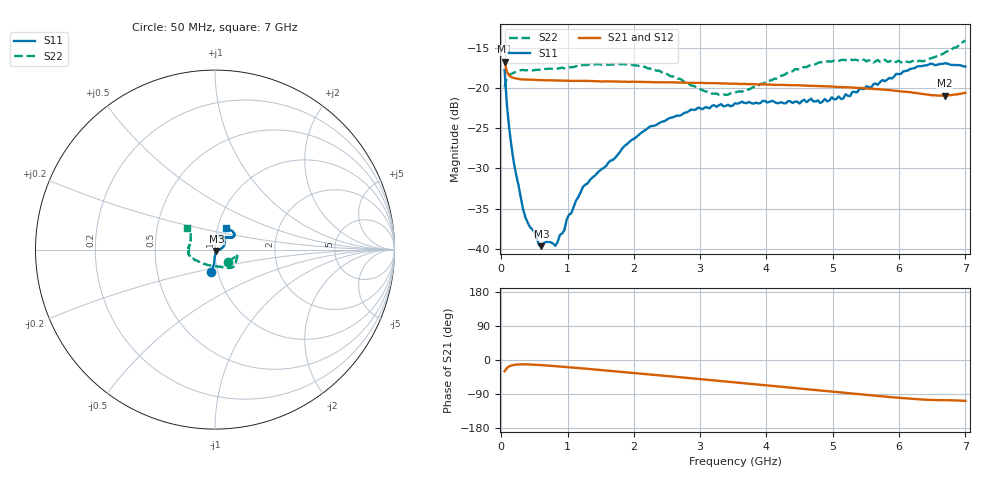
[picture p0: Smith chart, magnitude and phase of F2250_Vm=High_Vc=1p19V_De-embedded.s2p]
! Integrated Device Technology
! Corporate Headquarters
! 6024 Silver Creek Valley Road
! San Jose, CA 95138  USA
! Phone:  1-408-284-8200
! Toll Free:  1-800-223-1366
! Webpage:  http://www.idt.com/
! Timing and RF Division
! 515 Groton Road, Suite 102
! Westford, MA 01886-6024
! Device:  F2250
! Description: Voltage Variable RF Attenuator
! Frequency:  50.0 -  6000.00 MHz
! Package:  3x3 mm Thin QFN Plastic Package: 16 pin
! Ports:  2 RF, 3 DC
!  Pin  1  = GND
!  Pin  2  = NC
!  Pin  3  = RF1  = Port 1
!  Pin  4  = NC
!  Pin  5  = GND
!  Pin  6  = GND
!  Pin  7  = GND
!  Pin  8  = GND
!  Pin  9  = NC
!  Pin 10  = RF2  = Port 2
!  Pin 11  = NC
!  Pin 12  = GND
!  Pin 13  = GND
!  Pin 14  = VCNTRL
!  Pin 15  = VDD
!  Pin 16  = VMODE
! Vcntrl:  1.190 Volts
! Vmode:  +3.300 Volts
! Vdd:  +3.30  Volts
! Current:  1.330 mA
! Data:  The device was measured on a the F2250 evaluation board which has
!  individual transmission lines to the RF pins.  Data was collected
!  using a calibrated network analyzer.  The evaluation board was
!  de-embedded using a TRL calibration technique.
!  The reference plane is the edge of the package pin.
! Misc:  SN 10
!  Action Tracker AT0258
! Date Measured:  2014-11-26
! Date:  2015-10-15  MJV
! Note:
!  Integrated Device Technology supplies this data as a sample of measured
!  data at the package pin for this product.  Your particular data for this
!  product may vary.
!  Data was taken at 25 degrees C.
!  Integrated Device Technology reserves the right to change this data at anytime.
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# GHz S dB R 50
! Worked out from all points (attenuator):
!   201 points, 50 MHz to 7 GHz, reference 50 ohm
!   highest |S21| = -16.75 dB at 50 MHz (marker M1); lowest = -21.0 dB at 6.687 GHz (marker M2)
!   lowest |S11| = -39.6 dB at 606 MHz (marker M3), VSWR 1.02, Z = 50.7 - j0.741 ohm
!   |S11| at or under -10 dB: start of sweep to end of sweep
!   |S22| runs from -20.9 to -14.1 dB; largest |S21 - S12| = 0.00038
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0.05  -17.78 -99.8  -16.75 -29.8  -16.73 -29.8  -19.93 -42.3
0.08475  -22.13 -93.7  -18.02 -21.2  -18.02 -21.2  -18.62 -20.7
0.15425  -27.31 -92.7  -18.68 -14.4  -18.67 -14.4  -18.27 -13.0
0.189  -29.28 -90.4  -18.78 -13.0  -18.77 -13.0  -18.11 -12.4
0.328  -35.03 -76.1  -18.95 -11.4  -18.94 -11.4  -17.79 -12.8
0.43225  -37.28 -73.6  -18.98 -11.8  -19.00 -11.8  -17.83 -13.9
0.606  -39.64 -44.5  -19.04 -13.5  -19.06 -13.6  -17.70 -18.9
0.6755  -39.10 -40.2  -19.07 -14.4  -19.07 -14.4  -17.66 -20.3
0.8145  -39.61 -20.1  -19.08 -16.2  -19.09 -16.2  -17.65 -24.2
0.9535  -37.60 -23.2  -19.12 -18.1  -19.11 -18.2  -17.59 -27.9
0.98825  -36.28 -20.5  -19.12 -18.6  -19.12 -18.6  -17.54 -28.6
1.2315  -32.29 -4.4  -19.14 -22.3  -19.15 -22.3  -17.16 -33.8
1.857  -27.21 15.0  -19.23 -32.0  -19.24 -32.0  -17.07 -43.9
2.37825  -24.38 28.8  -19.31 -40.3  -19.29 -40.3  -17.85 -53.3
3.1775  -22.22 51.8  -19.43 -53.4  -19.42 -53.4  -20.72 -87.0
3.525  -21.93 62.7  -19.49 -59.1  -19.51 -59.1  -20.60 -111.2
4.7065  -21.68 67.7  -19.76 -78.7  -19.77 -78.7  -17.16 -161.1
5.15825  -21.32 51.0  -19.93 -86.3  -19.93 -86.3  -16.51 -170.2
5.85325  -18.78 36.1  -20.28 -97.7  -20.28 -97.8  -16.76 174.0
6.3745  -17.23 38.0  -20.77 -104.6  -20.77 -104.6  -16.70 156.3
6.68725  -16.97 45.7  -20.97 -106.0  -20.98 -106.2  -15.64 145.3
7  -17.36 62.1  -20.63 -107.9  -20.64 -107.9  -14.12 142.6
